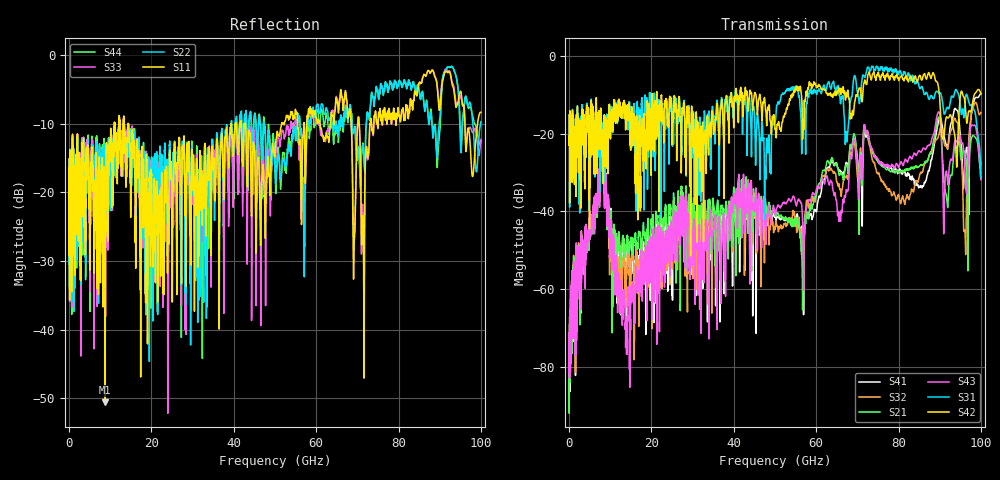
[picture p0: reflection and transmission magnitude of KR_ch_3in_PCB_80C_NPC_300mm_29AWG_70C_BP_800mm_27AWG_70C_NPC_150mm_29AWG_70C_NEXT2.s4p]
# Hz S RI R 45
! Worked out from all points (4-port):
!   4000 points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, 25 MHz to 100 GHz, reference 45 ohm
!   strongest paths, dB at 25 MHz, 25.02 GHz, 50.02 GHz, 75.03 GHz, 100 GHz:
!     S42: -20.7, -20.7, -18.8, -4.2, -9.7
!     S31: -20.7, -17.6, -16.6, -3.1, -31.3
!     S43: -82.8, -51.1, -40.5, -26.4, -31.8
!     S21: -81.6, -46.3, -40.4, -27.2, -27.3
!     S32: -84.3, -51.6, -44.7, -30.4, -14.5
!     S41: -90.0, -61.6, -41.2, -27.1, -9.7
!   lowest |S11| = -50.6 dB at 8.8 GHz (marker M1), VSWR 1.01, Z = 44.9 - j0.241 ohm
!   |S11| at or under -10 dB: start of sweep to 11.02 GHz; 13.41 GHz to 39.38 GHz (25.98 GHz wide, 98.4 % of centre); 42.86 GHz to 51.61 GHz (8.752 GHz wide, 18.5 % of centre)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
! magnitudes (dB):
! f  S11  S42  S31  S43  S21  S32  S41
! 25 MHz  -16.4  -20.7  -20.7  -82.8  -81.6  -84.3  -90.0
! 8.8 GHz  -50.6  -17.9  -23.5  -32.8  -32.7  -33.6  -32.2
! 14.38 GHz  -10.1  -14.3  -16.0  -61.1  -48.4  -51.3  -48.7
! 71.95 GHz  -15.3  -6.5  -5.3  -18.9  -19.4  -18.7  -20.0
! 93.95 GHz  -7.6  -24.6  -8.6  -21.9  -23.4  -16.7  -13.7
! 96.1 GHz  -9.6  -11.6  -13.3  -28.6  -24.7  -44.8  -27.3
! 100 GHz  -8.3  -9.7  -31.3  -31.8  -27.3  -14.5  -9.7
